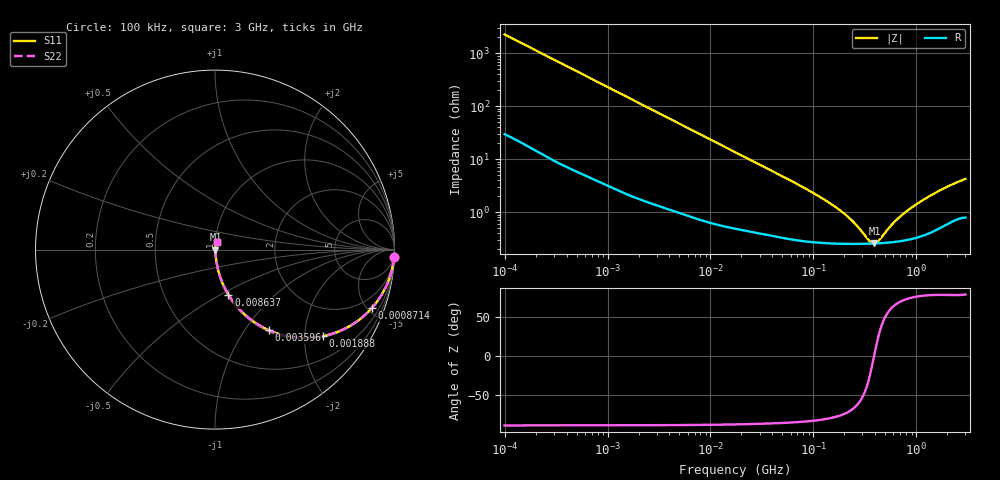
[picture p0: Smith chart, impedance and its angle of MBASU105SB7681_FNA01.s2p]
! MBASU105SB7681_FNA01  S-PARAMETER MODEL  ( Standard Model )
! Model Generated by TAIYO YUDEN Corporation (http://www.ty-top.com)
! Version 1.0
! TAIYO YUDEN Control No. 220601
! Copyright(c) 2017 TAIYO YUDEN CO.,LTD. All Rights Reserved.
! Product Description (link to TY-COMPAS)
! https://ds.yuden.co.jp/TYCOMPAS/or/detail?pn=MBASU105SB7681KFNA01&u=M
! Products Name : Multilayer Ceramic Capacitors
! Characteristics :
!  Capacitance : 680 [pF] , Rated Voltage : 50 [V] , TCC : X7R
!  Case Size : 1.0 x 0.5 / 0.039 x 0.02 [mm/inch] , Thickness : 0.5 / 0.02 [mm/inch]
!  (Conditions: Temperature = 25 [degC] , DC Bias Voltage = 0 [V])
! External Node Assignments :
!  1  o---| |---o  2
! GND o---------o GND
! Frequency Range : 100kHz  -  3GHz  [ 401 STEP ]
# MHZ S RI R 50
! Freq[MHz].  S11 Real  S11 Imag  S21 Real  S21 Imag  S12 Real  S12 Imag  S22 Real  S22 Imag
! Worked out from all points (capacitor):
!   401 points, 100 kHz to 3 GHz, reference 50 ohm
!   read as one part in series: C = 696 pF near 105.3 kHz
!   lowest |Z| = 255 mohm at 391.6 MHz (marker M1)
!   series resonance near 388.8 MHz, so ESL is about 240 pH
!   S11 on the Smith chart (normalised r, x): 100 kHz: 2, -46; 871.4 kHz: 1.07, -5.32; 1.888 MHz: 1.04, -2.47; 3.596 MHz: 1.02, -1.30; 8.637 MHz: 1.01, -0.55; 3 GHz: 1.02, +0.08
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0.1  0.9975 -0.0437  0.00249 0.0437  0.00249 0.0437  0.9975 -0.0437
0.259498  0.9861 -0.1111  0.0139 0.1111  0.0139 0.1111  0.9861 -0.1111
0.562235  0.9416 -0.2283  0.0584 0.2283  0.0584 0.2283  0.9416 -0.2283
0.871356  0.873 -0.3263  0.127 0.3263  0.127 0.3263  0.873 -0.3263
1.282589  0.7638 -0.4178  0.2362 0.4178  0.2362 0.4178  0.7638 -0.4178
1.887902  0.6028 -0.4819  0.3972 0.4819  0.3972 0.4819  0.6028 -0.4819
3.161081  0.3569 -0.4704  0.6431 0.4704  0.6431 0.4704  0.3569 -0.4704
3.595834  0.3018 -0.45  0.6982 0.45  0.6982 0.45  0.3018 -0.45
5.431059  0.1634 -0.3594  0.8366 0.3594  0.8366 0.3594  0.1634 -0.3594
8.636841  0.0751 -0.2515  0.9249 0.2515  0.9249 0.2515  0.0751 -0.2515
17.7727  0.0221 -0.1302  0.9779 0.1302  0.9779 0.1302  0.0221 -0.1302
97.38194  0.00325 -0.0233  0.9968 0.0233  0.9968 0.0233  0.00325 -0.0233
200.3904  0.00259 -0.00892  0.9974 0.00892  0.9974 0.00892  0.00259 -0.00892
259.3015  0.00253 -0.00522  0.9975 0.00522  0.9975 0.00522  0.00253 -0.00522
353.2796  0.00253 -0.0012  0.9975 0.0012  0.9975 0.0012  0.00253 -0.0012
391.6425  0.00255 9.15e-05  0.9975 -9.15e-05  0.9975 -9.15e-05  0.00255 9.15e-05
434.1712  0.00257 0.00139  0.9974 -0.00139  0.9974 -0.00139  0.00257 0.00139
547.5153  0.00268 0.00437  0.9973 -0.00437  0.9973 -0.00437  0.00268 0.00437
745.9503  0.00295 0.00872  0.9971 -0.00872  0.9971 -0.00872  0.00295 0.00872
1097.999  0.00367 0.0153  0.9963 -0.0153  0.9963 -0.0153  0.00367 0.0153
1886.474  0.0063 0.0277  0.9937 -0.0277  0.9937 -0.0277  0.0063 0.0277
3000  0.00955 0.0411  0.9905 -0.0411  0.9905 -0.0411  0.00955 0.0411
